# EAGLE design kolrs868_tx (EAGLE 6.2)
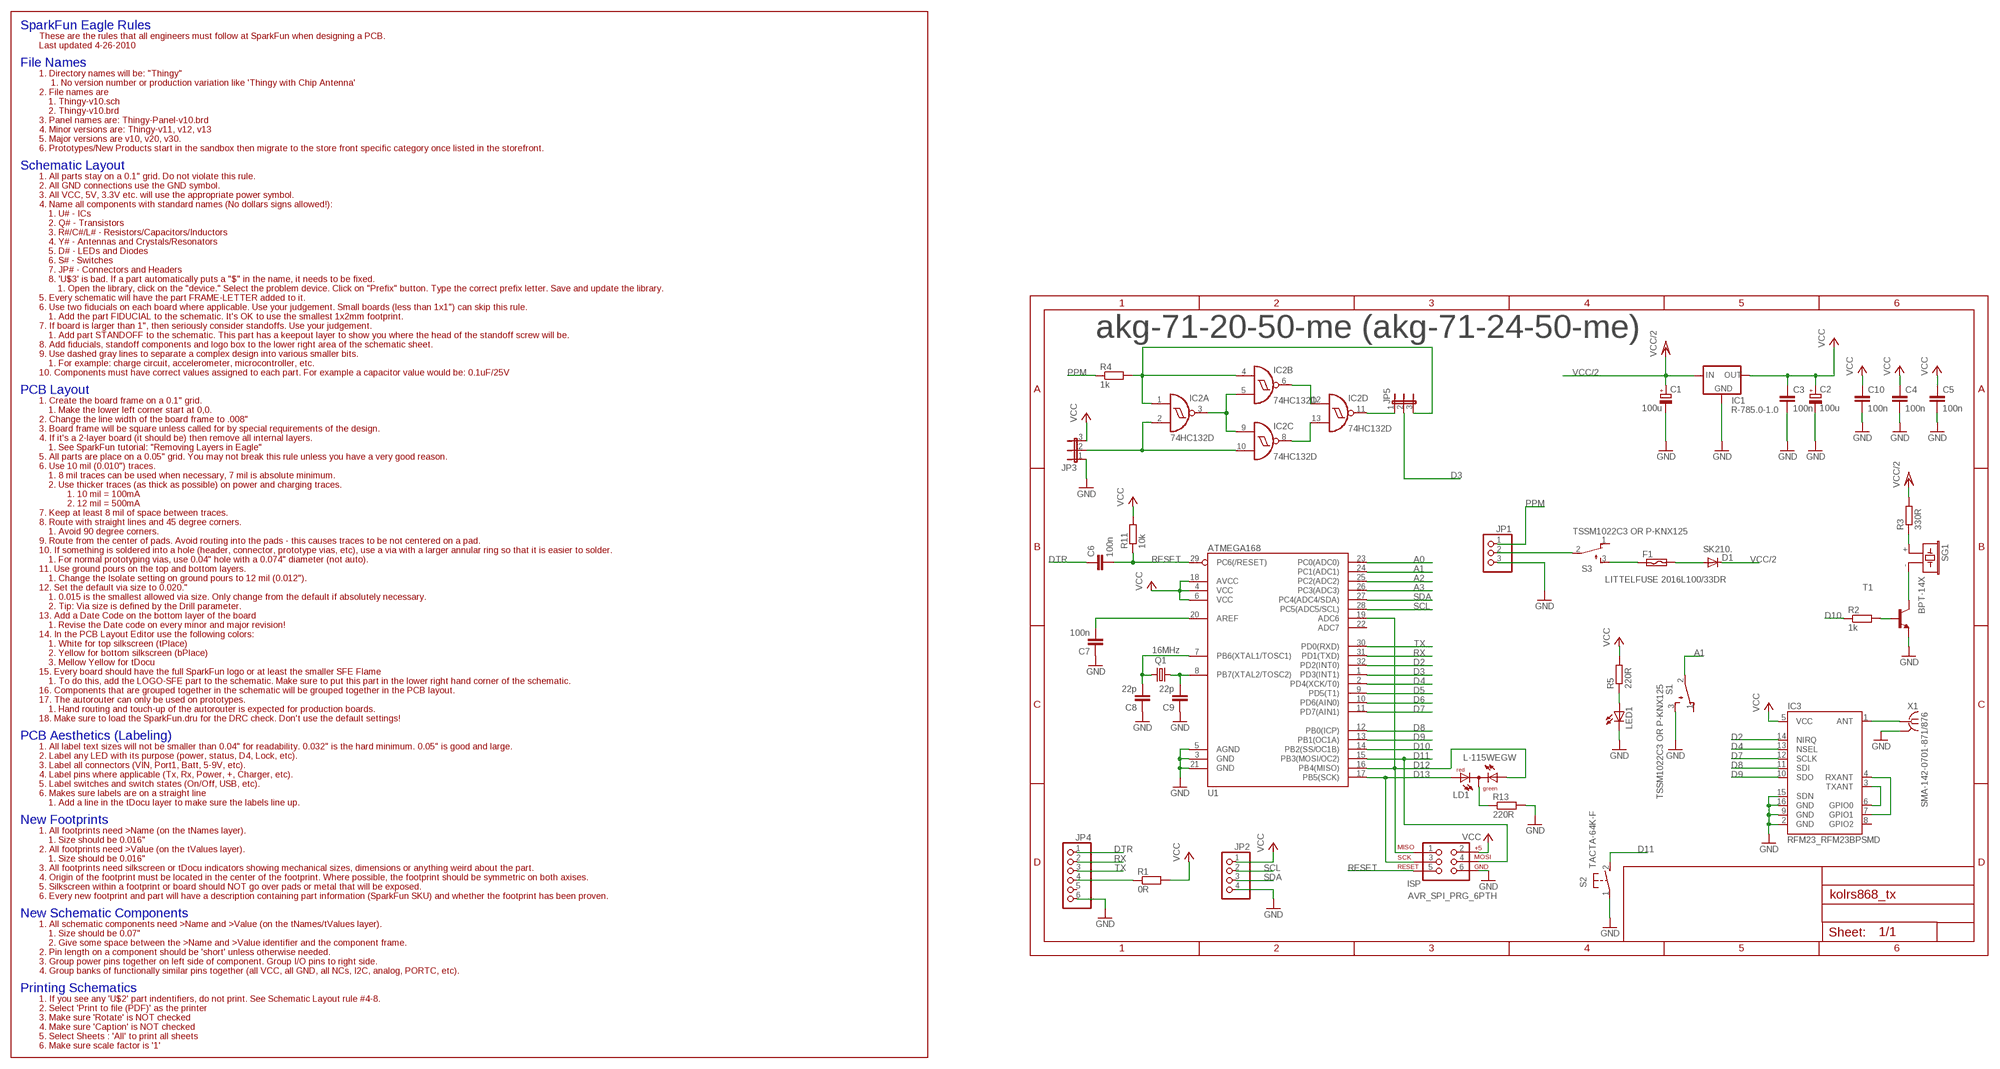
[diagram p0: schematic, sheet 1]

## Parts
C1  100u  CPOL-EUSMCB  [SMC_B]
C2  100u  CPOL-EUSMCB  [SMC_B]
C3  100n  C-EU_KOLIN  [M0805]
C4  100n  C-EU_KOLIN  [M0805]
C5  100n  C-EU_KOLIN  [M0805]
C6  100n  C-EU_KOLIN  [M0805]
C7  100n  C-EU_KOLIN  [M0805]
C8  22p  C-EU_KOLIN  [M0805]
C9  22p  C-EU_KOLIN  [M0805]
C10  100n  C-EU_KOLIN  [M0805]
D1  SK210.  DIODE-SMB  [SMB]
F1  LITTELFUSE 2016L100/33DR  SMD100F/33  [SMD050F]
IC1  R-785.0-1.0  78XX_RECOM  [78XX_RECOM]
IC2  74HC132D  [SO14]
IC3  RFM23_RFM23BPSMD  [RFM23_RFM23BP-S2]
ISP  AVR_SPI_PRG_6PTH  [2X3]
JP1  PINHD-1X3  [1X03]
JP2  PINHD-1X4  [1X04]
JP3  JP2E  [JP2]
JP4  PINHD-1X6  [1X06]
JP5  JP2E  [JP2]
LD1  L-115WEGW  DUOLED-RG-C  [DUOLED-C-5MM]
LED1  LED5MM  [LED5MM]
Q1  16MHz  CRYSTALHC49UP  [HC49UP]
R1  0R  R-EU_KOLINM0805  [M0805]
R2  1k  R-EU_KOLINM0805  [M0805]
R3  330R  R-EU_KOLINM0805  [M0805]
R4  1k  R-EU_KOLINM0805  [M0805]
R5  220R  R-EU_KOLINM0805  [M0805]
R11  10k  R-EU_KOLINM0805  [M0805]
R13  220R  R-EU_KOLINM0805  [M0805]
S1  TSSM1022C3 OR P-KNX125  TL32WO  [TL3XWO]
S2  TACTA-64K-F  31-XX  [B3F-31XX]
S3  TSSM1022C3 OR P-KNX125  TL32WO  [TL3XWO]
SG1  BPT-14X  F/CM12P  [F/CM12P]
T1  BC848-NPN-SOT23-BEC  [SOT23-BEC]
U1  ATMEGA168  [TQFP32-08]
X1  SMA-142-0701-871/876  [J502-ND-142-0701-871/876]

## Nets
A0: U1.23(PC0(ADC0))
A1: S1.2(P) U1.24(PC1(ADC1))
A2: U1.25(PC2(ADC2))
A3: U1.26(PC3(ADC3))
D2: IC3.14(NIRQ) U1.32(PD2(INT0))
D3: JP5.2 U1.1(PD3(INT1))
D4: IC3.13(NSEL) U1.2(PD4(XCK/T0))
D5: U1.9(PD5(T1))
D6: U1.10(PD6(AIN0))
D7: IC3.12(SCLK) U1.11(PD7(AIN1))
D8: IC3.11(SDI) U1.12(PB0(ICP))
D9: IC3.10(SDO) U1.13(PB1(OC1A))
D10: R2.1 U1.14(PB2(SS/OC1B))
D11: ISP.4 S2.2(S) U1.15(PB3(MOSI/OC2))
D12: ISP.1 LD1.AX(AG) U1.16(PB4(MISO)) U1.19(ADC6)
D13: ISP.3 LD1.AR U1.17(PB5(SCK))
DTR: C6.1 JP4.1
GND: C1.- C2.- C3.2 C4.2 C5.2 C7.1 C8.1 C9.1 C10.2 IC1.GND IC3.2(GND) IC3.9(GND) IC3.15(SDN) IC3.16(GND) ISP.6 JP1.3 JP2.4 JP3.1 JP4.6 LED1.K(C) R13.2 S1.3(S) S2.1(P) T1.E U1.3(GND) U1.5(AGND) U1.21(GND) X1.G@1(GND)
N$1: C7.2 U1.20(AREF)
N$2: IC3.3(TXANT) IC3.6(GPIO0)
N$3: IC3.4(RXANT) IC3.7(GPIO1)
N$4: IC3.1(ANT) X1.1
N$5: F1.1 S3.3(S)
N$6: C8.2 Q1.2 U1.7(PB6(XTAL1/TOSC1))
N$7: C9.2 Q1.1 U1.8(PB7(XTAL2/TOSC2))
N$8: LD1.C R13.1
N$9: D1.A F1.2
N$10: R2.2 T1.B
N$11: SG1.- T1.C
N$12: R3.1 SG1.+
N$13: JP1.2 S3.2(P)
N$14: LED1.A R5.1
N$15: JP4.4 R1.1
N$17: IC2.3(A:O) IC2.5(B:I1) IC2.9(C:I0)
N$18: IC2.11(D:O) JP5.1
N$19: IC2.2(A:I1) IC2.10(C:I1) JP3.2
N$20: IC2.8(C:O) IC2.13(D:I1)
N$21: IC2.6(B:O) IC2.12(D:I0)
N$24: IC2.1(A:I0) IC2.4(B:I0) JP5.3 R4.2
PPM: JP1.1 R4.1
RESET: C6.2 ISP.5 R11.1 U1.29(PC6(/RESET))
RX: JP4.2 U1.31(PD1(TXD))
SCL: JP2.2 U1.28(PC5(ADC5/SCL))
SDA: JP2.3 U1.27(PC4(ADC4/SDA))
TX: JP4.3 U1.30(PD0(RXD))
VCC: C2.+ C3.1 C4.1 C5.1 C10.1 IC1.OUT IC3.5(VCC) ISP.2 JP2.1 JP3.3 R1.2 R5.2 R11.2 U1.4(VCC) U1.6(VCC) U1.18(AVCC)
VCC/2: C1.+ D1.C IC1.IN R3.2
Unconnected: IC3.8(GPIO2) JP4.5 S1.1(O) S3.1(O) U1.22(ADC7)

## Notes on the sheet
- akg-71-20-50-me (akg-71-24-50-me)

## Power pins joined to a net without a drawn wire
GND: IC2.7(P:GND) X1.G@2(GND) X1.G@3(GND) X1.G@4(GND)
VCC: IC2.14(P:VCC)

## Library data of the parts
C1 C2 = rcl:CPOL-EU: POLARIZED CAPACITOR, European symbol
C3-C10 = PINHEAD_RC:C-EU_KOLIN: CAPACITOR, European symbol
D1 = diode:DIODE-: DIODE
F1 = switch-raychem:SMD*F: PolySwitch (TM) Resettable Device
IC1 = recom:78XX_RECOM: VOLTAGE REGULATOR
IC2 = 74xx-eu:74*132: Quad 2-input NAND schmitt trigger
IC3 = openLRSngTX:RFM23_RFM23BP: The RFM23BP is a medium power, low cost radio that is capable of operating in the 434MHz and 900MHz open bands. It s frequency is software defined and there are some very good libraries written for it.'
ISP = SparkFun:AVR_SPI_PRG_6: AVR ISP 6 Pin This is the reduced ISP connector for AVR programming. Common on Arduino. This footprint will take up less PCB space and can be used with a 10-pin to 6-pin adapter such as SKU: BOB-08508
JP1 = pinhead:PINHD-1X3: PIN HEADER
JP2 = pinhead:PINHD-1X4: PIN HEADER
JP3 JP5 = jumper:JP2E: JUMPER
JP4 = pinhead:PINHD-1X6: PIN HEADER
LD1 = led:DUOLED-RG-C: DUO LED 2 colors (red/green), 5 mm, round, common Cathode www.ligitek.com or other producers.
LED1 = led:LED: LED
Q1 = crystal:CRYSTAL: CRYSTAL; OC_FARNELL: unknown; OC_NEWARK: unknown
R1-R5 R11 R13 = PINHEAD_RC:R-EU_KOLIN: RESISTOR, European symbol
S1 S3 = switch:TL32WO: TINY SWITCH ON - MOM Source: http://www2.produktinfo.conrad.com/datenblaetter/700000-724999/705152-da-01-de-Subminiaturschalter_TL_36WO.pdf
S2 = switch-omron:31-XX: OMRON SWITCH; MPN: B3F-3100; OC_FARNELL: 959704; OC_NEWARK: 36M3582
SG1 = buzzer:F/CM12P: BUZZER; OC_FARNELL: unknown; OC_NEWARK: unknown
T1 = transistor:*-NPN-: NPN Transistror BF959 corrected 2008.03.06
U1 = SparkFun:ATMEGA168
X1 = con-coax:SMA-: SMA 50 Ohm End Launch Jack Receptacle - Round Contact Johnson Components Source: www.johnsoncomponents.com .. J502-ND.pdf; MF: JOHNSON COMPONENTS; MPN: 142-0701-871; OC_FARNELL: 1339835; OC_NEWARK: 91B6105

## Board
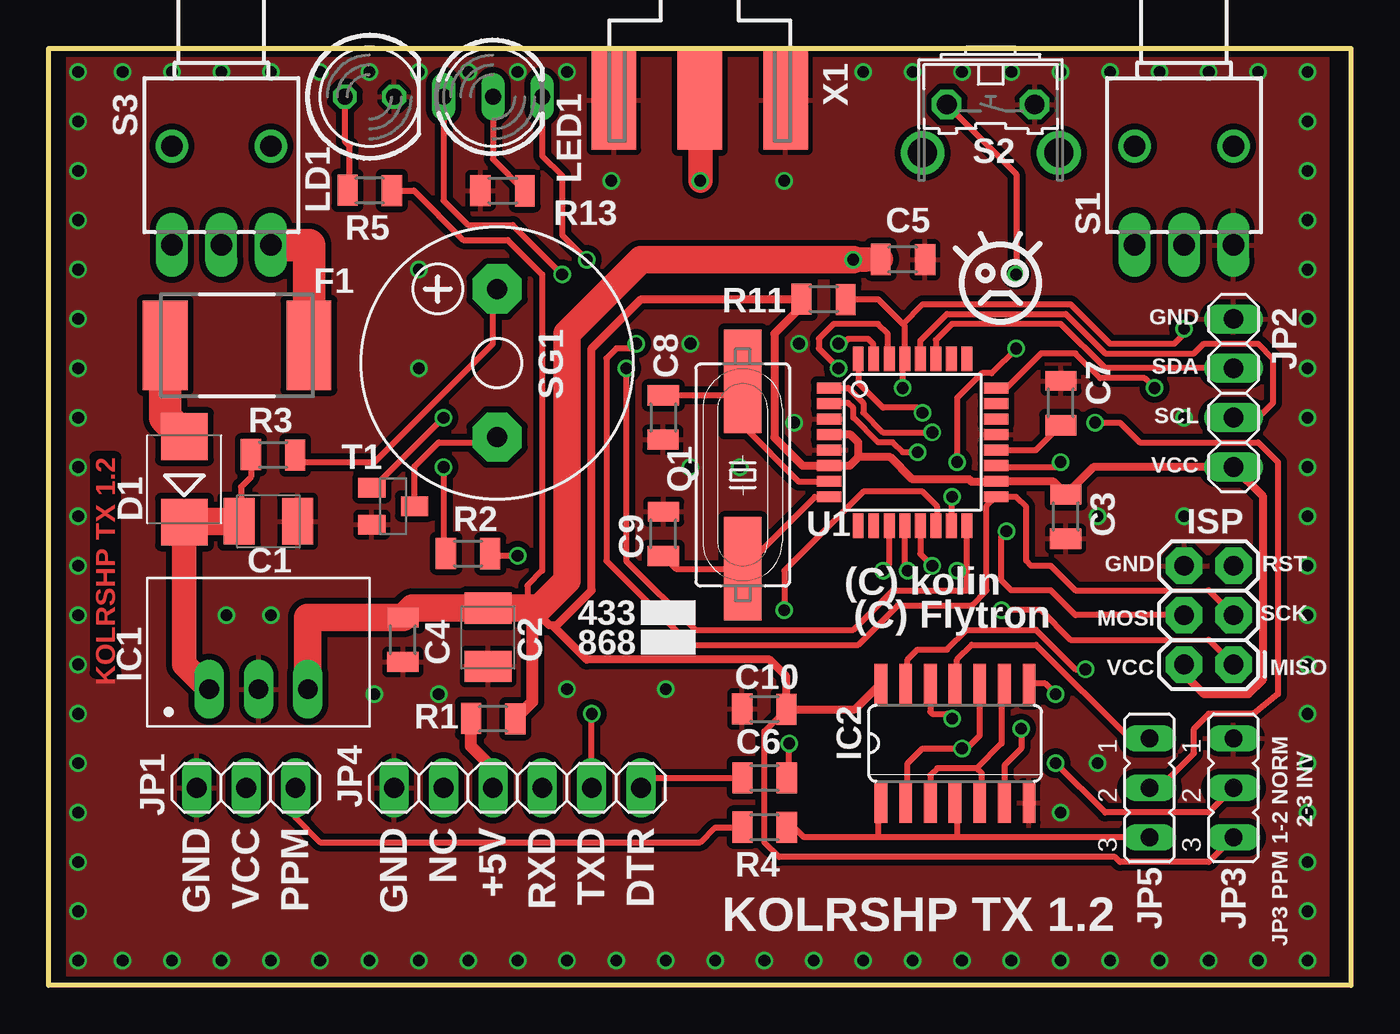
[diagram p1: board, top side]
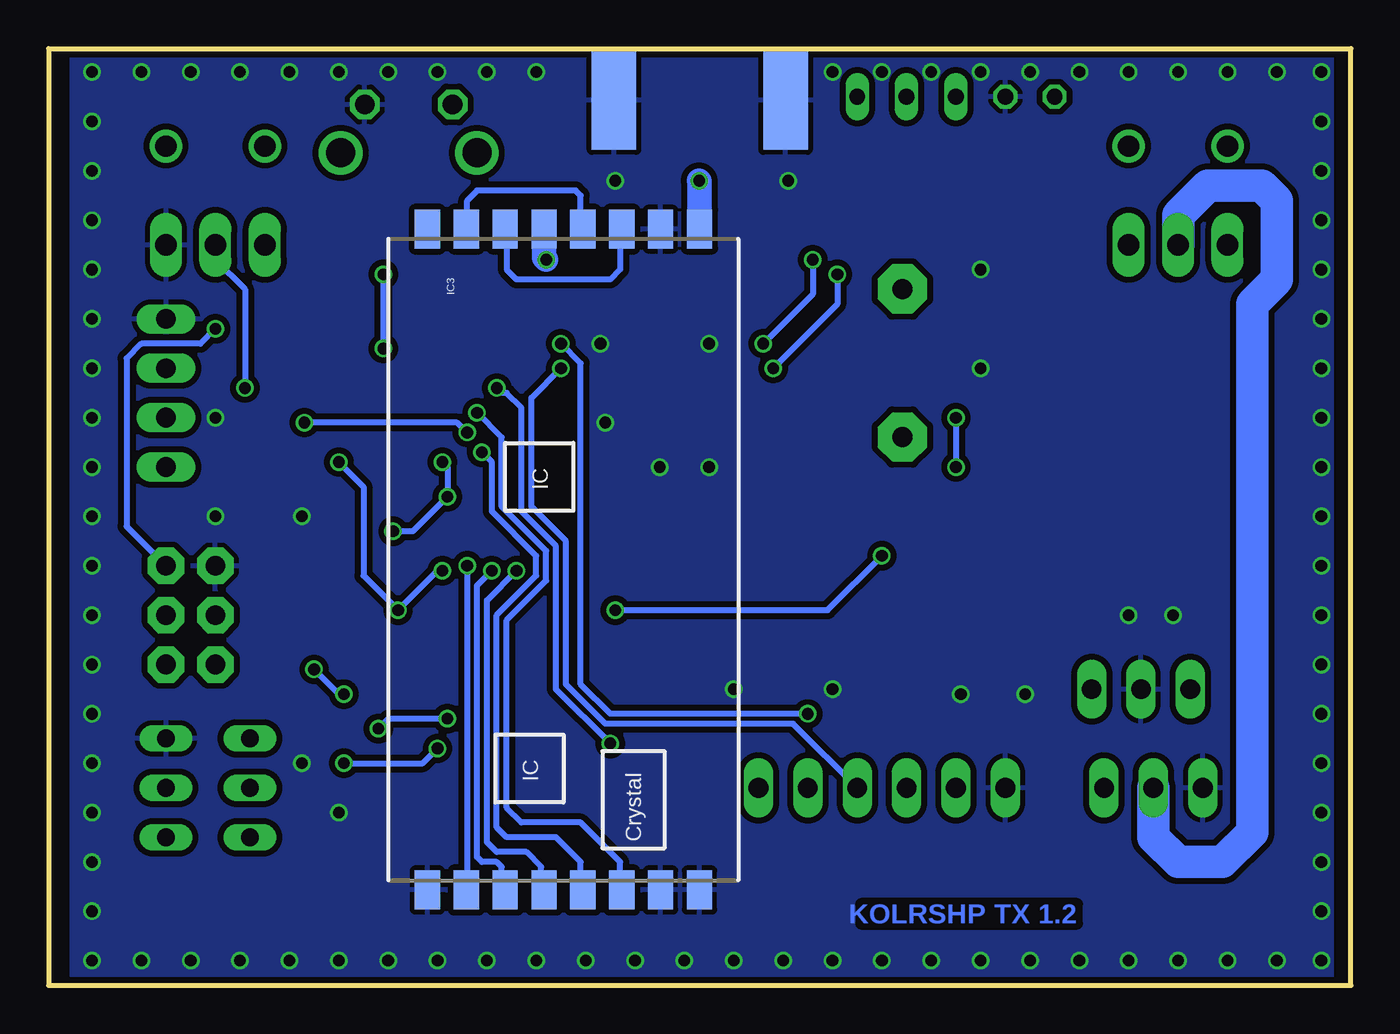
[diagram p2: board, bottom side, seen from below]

Size 67 x 48.2 mm. Coordinates in mm from the lower left corner, seen from the top.
Outline: 67,48.2 0,48.2 0,0 67,0 67,48.2
Copper layers (1*16): Top 0.018mm / dielectric 1.5mm / Bottom 0.018mm
Design rules: minimum track width 0.21mm, minimum drill 0.5mm, track to track 0.2mm, track to pad 0.2mm, pad to pad 0.2mm, via to via 0.2mm, smd to smd 0.2mm, copper to edge 10mil, drill to drill 8mil, minimum pad ring 0.15mm, minimum via ring 0.15mm, stop-mask expansion 4mil, vias tented up to drill 1mm, thermal gap 10mil

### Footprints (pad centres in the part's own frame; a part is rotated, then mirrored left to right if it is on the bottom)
SMC_B = smd 1.6 x 2.4: + -1.5,0; - 1.5,0
M0805 = smd 1.021 x 1.6: 1 -1.131,0.017 | smd 1.046 x 1.6: 2 1.148,0
SMB = smd 2.4 x 2.4: A 2.2,0; C -2.2,0
SMD050F = smd 2.3 x 4.6: 1 -3.7,0; 2 3.7,0
78XX_RECOM = drill 1.016 long: GND 0,-2.54; IN -2.54,-2.54; OUT 2.54,-2.54
SO14 = smd 0.66 x 2.032: 1 -3.81,-3.073; 2 -2.54,-3.073; 3 -1.27,-3.073; 4 0,-3.073; 5 1.27,-3.073; 6 2.54,-3.073; 7 3.81,-3.073; 8 3.81,3.073; 9 2.54,3.073; 10 1.27,3.073; 11 0,3.073; 12 -1.27,3.073; 13 -2.54,3.073; 14 -3.81,3.073
RFM23_RFM23BP-S2 = smd 2 x 1.3: 1 -17,7; 2 -17,5; 3 -17,3; 4 -17,1; 5 -17,-1; 6 -17,-3; 7 -17,-5; 8 -17,-7; 9 17,-7; 10 17,-5; 11 17,-3; 12 17,-1; 13 17,1; 14 17,3; 15 17,5; 16 17,7
2X3 = drill 1.016 pad 1.88 octagon: 1 0,0; 2 0,2.54; 3 2.54,0; 4 2.54,2.54; 5 5.08,0; 6 5.08,2.54
1X03 = drill 1.016 long: 1 -2.54,0; 2 0,0; 3 2.54,0
1X04 = drill 1.016 long: 1 -3.81,0; 2 -1.27,0; 3 1.27,0; 4 3.81,0
JP2 = drill 0.914 long: 1 -2.54,0; 2 0,0; 3 2.54,0
1X06 = drill 1.016 long: 1 -6.35,0; 2 -3.81,0; 3 -1.27,0; 4 1.27,0; 5 3.81,0; 6 6.35,0
DUOLED-C-5MM = drill 0.813 long: AR 2.54,0; AX -2.54,0; C 0,0
LED5MM = drill 0.813 octagon: A -1.27,0; K 1.27,0
HC49UP = smd 5.334 x 1.93: 1 -4.826,0; 2 4.826,0
TL3XWO = drill 1.1 pad 1.422 long: 1 -2.54,-5.08; 2 0,-5.08; 3 2.54,-5.08 | drill 1.1 pad 1.676: M1 -2.54,0; M2 2.54,0
B3F-31XX = drill 1.016 octagon: 1 -2.261,-1.245; 2 2.261,-1.245 | drill 1.499 pad 2.159: 3 -3.505,1.245; 4 3.505,1.245
F/CM12P = drill 1.016 pad 2.54 octagon: + 3.81,0; - -3.81,0
SOT23-BEC = smd 1 x 1.4: B -0.95,-1.1; C 0,1.1; E 0.95,-1.1
TQFP32-08 = smd 1.27 x 0.559: 1 -4.293,2.8; 2 -4.293,2; 3 -4.293,1.2; 4 -4.293,0.4; 5 -4.293,-0.4; 6 -4.293,-1.2; 7 -4.293,-2; 8 -4.293,-2.8; 17 4.293,-2.8; 18 4.293,-2; 19 4.293,-1.2; 20 4.293,-0.4; 21 4.293,0.4; 22 4.293,1.2; 23 4.293,2; 24 4.293,2.8 | smd 0.559 x 1.27: 9 -2.8,-4.293; 10 -2,-4.293; 11 -1.2,-4.293; 12 -0.4,-4.293; 13 0.4,-4.293; 14 1.2,-4.293; 15 2,-4.293; 16 2.8,-4.293; 25 2.8,4.293; 26 2,4.293; 27 1.2,4.293; 28 0.4,4.293; 29 -0.4,4.293; 30 -1.2,4.293; 31 -2,4.293; 32 -2.8,4.293
J502-ND-142-0701-871/876 = smd 5.08 x 2.286: 1 2.565,0; G@1 2.565,4.42; G@2 2.565,-4.42 | smd 5.08 x 2.286 bottom: G@3 2.565,4.42; G@4 2.565,-4.42

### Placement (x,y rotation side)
C1  11.3,23.88 0 top
C2  22.61,17.91 270 top
C3  52.32,24.13 270 top
C4  18.23,17.79 270 top
C5  43.94,37.34 0 top
C6  36.83,10.67 0 top
C7  52.07,29.97 270 top
C8  31.62,29.21 90 top
C9  31.62,23.24 270 top
C10  36.83,14.22 180 top
D1  6.99,26.04 90 top
F1  9.69,32.93 180 top
IC1  10.79,17.78 0 top
IC2  46.63,12.46 0 top
IC3  40.51,21.91 270 bottom
ISP  60.96,16.51 90 top
JP1  10.16,10.16 180 top
JP2  60.96,30.48 90 top
JP3  60.96,10.16 270 top
JP4  24.13,10.16 180 top
JP5  56.64,10.16 270 top
LD1  22.86,45.72 0 top
LED1  16.51,45.72 0 top
Q1  35.71,26.26 90 top
R1  22.86,13.72 0 top
R2  21.59,22.23 180 top
R3  11.56,27.3 180 top
R4  36.83,8.13 0 top
R5  16.51,40.89 0 top
R11  39.88,35.31 180 top
R13  23.37,40.89 180 top
S1  58.42,43.18 0 top
S2  48.47,44.08 180 top
S3  8.89,43.18 0 top
SG1  23.07,32.02 90 top
T1  17.73,24.66 270 top
U1  44.45,27.94 0 top
X1  33.5,48.1 270 top

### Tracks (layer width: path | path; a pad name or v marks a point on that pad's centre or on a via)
A1  (via drill 0.6)
  Top 0.305: v56.9,30.73 56.39,31.24 54.1,31.24 52.83,32.51 51.05,32.51 49.28,30.73 48.77,30.73 U1.24
  Bottom 0.305: v56.9,30.73 56.9,35.81 58.42,37.34 S1.2
D2  (via drill 0.6)
  Top 0.305: v44.96,29.46 44.7,29.72 42.93,29.72 41.66,30.99 41.66,32 U1.32
  Bottom 0.305: IC3.14 37.59,4.99 37.59,6.35 39.62,8.38 42.67,8.38 43.43,9.14 43.43,18.8 41.4,20.83 41.4,22.35 43.69,24.64 43.69,28.19 v44.96,29.46
D3  (via drill 0.6)
  Top 0.305: U1.1 41.14,30.74 41.91,29.97 41.91,29.46 42.93,28.45 v45.47,28.45 | v53.85,28.96 55.12,28.96 56.13,27.94 62.23,27.94 63.25,26.92 63.25,14.99 61.98,13.97 59.69,13.97 58.93,13.21 58.93,11.94 57.15,10.16 JP5.2
  Bottom 0.305: v53.85,28.96 45.97,28.96 v45.47,28.45
D4  (via drill 0.6)
  Top 0.305: v44.7,27.43 43.94,27.43 43.43,27.94 42.67,27.94 41.4,29.21 41.4,29.72 41.15,29.97 40.19,29.97 U1.2
  Bottom 0.305: IC3.13 39.62,5.02 39.62,6.35 40.89,7.62 43.43,7.62 43.94,8.13 43.94,19.05 41.91,21.08 41.91,22.1 44.2,24.38 44.2,26.92 v44.7,27.43
D7  (via drill 0.6)
  Top 0.305: v42.93,21.34 43.25,21.66 U1.11
  Bottom 0.305: IC3.12 41.66,5.05 41.66,6.1 42.42,6.86 43.94,6.86 44.45,7.37 44.45,19.81 v42.93,21.34
D8  (via drill 0.6)
  Top 0.305: v44.2,21.34 44.05,21.48 U1.12
  Bottom 0.305: IC3.11 43.69,5.08 43.69,6.1 43.94,6.35 44.7,6.35 44.96,6.6 44.96,20.57 v44.2,21.34
D9  (via drill 0.6)
  Top 0.305: U1.13 44.85,22.21 v45.47,21.59
  Bottom 0.305: v45.47,21.59 45.47,4.96 IC3.10
D10  (via drill 0.6)
  Top 0.305: v37.85,19.3 37.85,21.34 41.91,25.4 44.96,25.4 45.72,24.64 45.72,23.88 U1.14 | v24.13,22.1 22.83,22.1 R2.1
  Bottom 0.305: v37.85,19.3 26.92,19.3 v24.13,22.1
D11  (via drill 0.6)
  Top 0.305: S2.2 49.78,41.75 v49.78,36.58 | v49.78,32.77 48.51,31.5 48.01,31.5 46.74,30.23 v46.74,26.92 | v46.48,25.15 46.45,25.11 U1.15 | ISP.4 52.83,19.05 51.56,20.32 49.53,20.32 49.02,20.83 49.02,23.11 v49.28,23.37
  Bottom 0.305: v49.78,36.58 v49.78,32.77 | v46.74,26.92 46.48,26.67 v46.48,25.15 48.26,23.37 v49.28,23.37
D12  (via drill 0.6)
  Top 0.254: 57.66,17.78 59.69,17.78
  Top 0.305: LD1.AX 20.32,40.39 21.59,39.12 23.88,39.12 v26.42,36.58 | U1.16 47.25,21.34 | v29.72,31.75 29.72,21.84 33.27,18.29 41.4,18.29 43.43,20.32 47.24,20.32 47.25,20.33 47.25,21.34 | ISP.1 59.69,17.78 | v49.02,19.3 51.05,19.3 52.58,17.78 57.66,17.78 | v46.74,21.34 47.25,21.34 | v52.07,26.92 52.07,26.67 48.26,26.67 U1.19
  Bottom 0.305: v26.42,36.58 26.42,35.05 v29.72,31.75 | v46.74,21.34 46.99,21.34 v49.02,19.3 50.8,21.08 50.8,25.65 v52.07,26.92
D13  (via drill 0.6)
  Top 0.254: 57.66,20.32 59.69,20.32
  Top 0.305: LD1.AR 25.4,42.67 26.42,41.66 26.42,38.61 v27.69,37.34 | v30.23,33.02 29.97,32.77 29.21,32.77 28.7,32.26 28.7,21.84 33.02,17.53 41.66,17.53 43.69,19.56 47.5,19.56 48.26,20.32 48.26,24.66 U1.17 49.79,25.14 50.29,24.64 50.29,21.84 50.55,21.59 51.56,21.59 52.83,20.32 57.66,20.32 | ISP.3 59.82,20.19 59.69,20.32
  Bottom 0.305: v27.69,37.34 27.69,35.56 v30.23,33.02
DTR
  Top 0.305: JP4.1 31,10.69 C6.1
GND  (via drill 0.6)
  other vias: 11.43,19.05 19.05,36.83 19.05,31.75 54.61,46.99 3.81,1.27 6.35,1.27 8.89,1.27 11.43,1.27 13.97,1.27 16.51,1.27 19.05,1.27 21.59,1.27 24.13,1.27 26.67,1.27 29.21,1.27 31.75,1.27 34.29,1.27 36.83,1.27 39.37,1.27 41.91,1.27 44.45,1.27 46.99,1.27 49.53,1.27 52.07,1.27 54.61,1.27 57.15,1.27 59.69,1.27 62.23,1.27 64.77,24.13 64.77,26.67 64.77,1.27 64.77,3.81 64.77,6.35 64.77,8.89 64.77,11.43 64.77,13.97 64.77,16.51 64.77,24.13 52.07,46.99 49.53,46.99 46.99,46.99 44.45,46.99 41.91,46.99 24.13,46.99 26.67,46.99 1.52,1.27 1.52,3.81 1.52,6.35 1.52,8.89 1.52,11.43 1.52,13.97 1.52,16.51 1.52,19.05 1.52,21.59 1.52,24.13 1.52,26.67 1.52,29.21 1.52,31.75 1.52,34.29 1.52,36.83 1.52,39.37 1.52,41.91 1.52,44.45 1.52,46.99 3.81,46.99 6.35,46.99 8.89,46.99 11.43,46.99 13.97,46.99 16.51,46.99 19.05,46.99 21.59,46.99 31.75,15.24 26.67,15.24 52.07,8.89 57.15,46.99 59.69,46.99 62.23,46.99 64.77,46.99 64.77,44.45 64.77,41.91 64.77,39.37 64.77,36.83 64.77,34.29 64.77,31.75 64.77,29.21 64.77,21.59 64.77,19.05 33.02,33.02 33.02,26.67 35.56,26.67 58.42,29.21 58.42,24.13 38.61,33.02 38.35,28.96 37.85,41.4 28.96,41.4 53.98,24.13 53.98,11.43 9.14,19.05 20.07,14.99 16.76,14.99
  pour Bottom (isolate 0.305): 1.02,0.25 65.79,0.51 65.79,48.01 1.02,48.01
  pour Top (isolate 0.305): 1.02,0.25 65.79,0.51 65.79,48.01 1.02,48.01
N$1
  Top 0.305: U1.20 50.79,27.54 C7.2
N$2
  Bottom 0.305: IC3.3 37.59,38.86 37.59,36.83 38.1,36.32 42.93,36.32 43.43,36.83 43.43,38.86 IC3.6
N$3
  Bottom 0.305: IC3.4 39.62,39.12 39.62,40.64 39.88,40.89 44.96,40.89 45.47,40.39 45.47,39.12 IC3.7
N$4  (via drill 0.6)
  Top 1.27: v33.53,41.4 33.53,45.51 X1.1
  Bottom 1.27: IC3.1 33.51,41.39 v33.53,41.4
N$5
  Top 1.676: S3.3 13.39,38.1 F1.1
N$6
  Top 0.305: C8.2 34.99,30.36 Q1.2 35.71,28.8 38.61,25.91 40.12,25.91 U1.7
N$7
  Top 0.305: C9.2 32.28,21.43 Q1.1 39.42,25.14 U1.8
N$8
  Top 0.305: LD1.C 22.86,42.52 R13.1
N$9
  Top 1.676: F1.2 5.99,29.23 D1.A
N$10  (via drill 0.6)
  Top 0.305: v20.32,26.67 20.32,22.86 R2.2 | v20.32,29.21 16.51,25.4 T1.B
  Bottom 0.305: v20.32,29.21 v20.32,26.67
N$11
  Top 0.305: T1.C 18.83,26.7 20.07,27.94 22.8,27.94 SG1.-
N$12
  Top 0.305: R3.1 12.45,27.18 12.7,26.92 16.76,26.92 22.86,33.02 22.86,35.81 SG1.+
N$13
  Bottom 1.676: JP1.2 10.16,7.62 8.89,6.35 6.6,6.35 5.08,7.87 5.08,35.05 3.81,36.32 3.81,40.39 4.57,41.15 7.37,41.15 8.89,39.62 S3.2
N$14
  Top 0.305: R5.1 15.49,41.15 15.49,43.18 15.24,43.43 LED1.A
N$15
  Top 0.61: JP4.4 22.86,11.18 21.73,12.31 R1.1
N$17
  Top 0.305: IC2.5 48.01,9.49 48.01,10.92 47.75,11.18 | 47.75,11.18 45.72,11.18 45.36,10.82 IC2.3 | IC2.9 49.02,15.38 49.02,12.45 47.75,11.18
N$18
  Top 0.305: IC2.11 46.74,15.64 46.74,16.76 47.5,17.53 50.8,17.53 55.63,12.7 JP5.1
N$19  (via drill 0.6)
  Top 0.305: IC2.2 44.2,9.49 44.2,11.43 44.96,12.19 v46.99,12.19 47.24,12.19 47.37,12.32 47.9,12.85 IC2.10 | JP3.2 59.69,8.89 54.36,8.89 v51.82,11.43
  Bottom 0.305: v51.82,11.43 47.75,11.43 v46.99,12.19
N$20  (via drill 0.6)
  Top 0.305: IC2.13 44.2,15.64 44.2,16.76 44.7,17.27 46.23,17.27 47.24,18.29 50.8,18.29 52.83,16.26 v53.34,16.26 | v51.82,14.99 51.27,15.53 IC2.8
  Bottom 0.305: v53.34,16.26 52.07,14.99 v51.82,14.99
N$21  (via drill 0.6)
  Top 0.305: IC2.12 45.36,14.07 45.47,13.97 46.23,13.97 v46.48,13.72 | v50.04,13.21 50.04,12.19 49.17,11.33 IC2.6
  Bottom 0.305: v46.48,13.72 49.53,13.72 v50.04,13.21
N$24
  Top 0.305: JP5.3 46.74,7.62 | 46.74,7.62 42.67,7.62 | 42.67,7.62 38.86,7.62 38.35,8.13 R4.2 | IC2.1 42.67,9.24 42.67,7.62 | IC2.4 46.74,9.28 46.74,7.62
PPM
  Top 0.305: JP1.1 12.7,8.64 13.97,7.37 33.53,7.37 34.29,8.13 35.68,8.13 R4.1
RESET  (via drill 0.6)
  Top 0.305: 37.96,10.69 C6.2 38.1,10.67 v38.1,12.45 | 43.94,34.04 44.05,33.93 U1.29 43.94,32 v43.94,30.73 | 43.94,34.04 42.69,35.29 R11.1 | 43.94,34.04 44.96,35.05 52.58,35.05 54.61,33.02 57.91,33.02 58.42,33.53 v58.42,33.78
  Bottom 0.305: v58.42,33.78 59.18,33.02 62.23,33.02 62.99,32.26 62.99,23.62 ISP.5 | v43.94,30.73 43.69,30.48 43.43,30.48 42.67,29.72 42.67,24.38 40.89,22.61 40.89,15.24 v38.1,12.45
RX  (via drill 0.6)
  Top 0.305: v40.64,33.02 40.89,33.02 41.15,33.27 42.16,33.27 42.42,33.02 42.42,32.26 U1.31 | JP4.2 v27.94,13.97
  Bottom 0.305: v40.64,33.02 39.62,32 39.62,15.49 38.1,13.97 v27.94,13.97
SCL
  Top 0.305: U1.28 44.85,33.17 46.23,34.54 52.32,34.54 54.36,32.51 58.93,32.51 59.44,33.02 62.23,33.02 62.99,32.26 62.99,29.97 62.23,29.21 JP2.2
SDA
  Top 0.305: JP2.3 54.36,31.75 52.07,34.04 46.48,34.04 45.65,33.2 U1.27
TX  (via drill 0.6)
  Top 0.305: v40.64,31.75 39.62,32.77 39.62,33.27 40.39,34.04 42.67,34.04 43.18,33.53 43.18,32.26 U1.30
  Bottom 0.305: v40.64,31.75 42.16,30.23 42.16,24.64 40.39,22.86 40.39,15.49 38.35,13.46 28.7,13.46 JP4.3
VCC  (via drill 0.6)
  Top 0.305: R5.2 18.8,40.89 21.34,38.35 23.62,38.35 25.4,36.58 25.4,21.34 24.64,20.57 24.64,19.41 | JP3.3 59.69,6.35 55.12,6.35 54.86,6.6 37.59,6.6 36.83,7.37 36.83,13.08 C10.1
  Top 0.406: ISP.2 58.42,16 59.44,14.99 61.72,14.99 62.48,15.75 62.48,25.15 JP2.1 53.75,26.67 C3.1 51.66,25.94 U1.18 48.71,25.91 47.5,25.91 47.37,26.04 44.45,26.04 43.31,27.18 41.66,27.18 | 24.89,19.41 25.76,18.54 25.91,18.54 | 25.91,18.54 26.16,18.54 27.94,20.32 27.94,32.77 30.48,35.31 R11.2 38.86,35.17 38.86,35.05 37.34,33.53 37.34,28.19 38.79,26.74 U1.6 41.22,26.74 41.66,27.18 | 41.66,27.18 41.66,27.94 41.26,28.34 U1.4 | IC2.14 41.5,14.21 C10.1 37.96,15.89 37.08,16.76 27.69,16.76 25.91,18.54
  Top 0.61: R1.2 24.89,14.6 24.89,19.41
  Top 1.27: C5.1 42.03,37.34 v41.4,37.34
  Top 1.422: v41.4,37.34 30.48,37.34 26.67,33.53 26.67,20.83 25.25,19.41 24.89,19.41 24.64,19.41 C2.+ 18.73,19.41 C4.1 13.34,18.92 IC1.OUT
  Bottom 1.27: IC3.5 41.51,37.45 v41.4,37.34
VCC/2
  Top 0.305: C1.+ 9.91,23.88 9.91,25.65 10.41,26.16 10.41,27.18 R3.2
  Top 1.27: D1.C 6.99,16.51 IC1.IN
  Top 1.422: C1.+ 7.37,23.88 D1.C

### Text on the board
Top: KOLRSHP TX 1.2
Bottom: KOLRSHP TX 1.2
tPlace: GND | SDA | SCL | VCC | (C) kolin | GND | RST | 433 | (C) Flytron | SCK | MOSI | 868 | VCC | MISO | GND | VCC | PPM | GND | NC | +5V | RXD | TXD | DTR | 2-3 INV | KOLRSHP TX 1.2 | JP3 PPM 1-2 NORM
